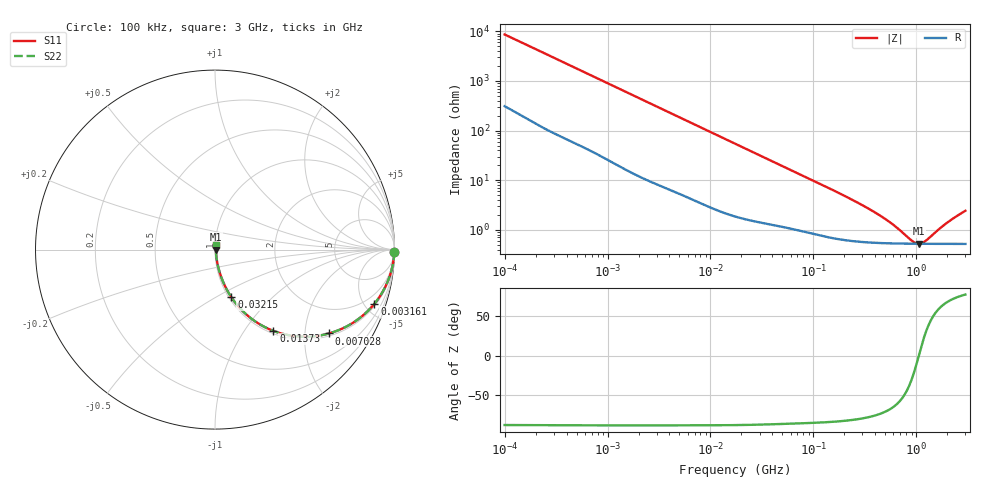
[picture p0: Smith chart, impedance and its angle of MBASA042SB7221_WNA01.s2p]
! MBASA042SB7221_WNA01  S-PARAMETER MODEL  ( Standard Model )
! Model Generated by TAIYO YUDEN Corporation (https://www.yuden.co.jp/en/)
! Version 1.0
! TAIYO YUDEN Control No. 250312
! Copyright(c) 2025 TAIYO YUDEN CO.,LTD. All Rights Reserved.
! Product Description (link to TY-COMPAS)
! https://ds.yuden.co.jp/TYCOMPAS/or/detail?pn=MBASA042SB7221KWNA01&u=M
! Products Name : Multilayer Ceramic Capacitors
! Characteristics :
!  Capacitance : 220 [pF] , Rated Voltage : 4 [V] , TCC : X7R
!  Case Size : 0.4 x 0.2 / 0.016 x 0.008 [mm/inch] , Thickness : 0.2 / 0.008 [mm/inch]
!  (Conditions: Temperature = 25 [degC] , DC Bias Voltage = 0 [V])
! External Node Assignments :
!  1  o---| |---o  2
! GND o---------o GND
! Frequency Range : 100kHz  -  3GHz  [ 401 STEP ]
# MHZ S RI R 50
! Freq[MHz].  S11 Real  S11 Imag  S21 Real  S21 Imag  S12 Real  S12 Imag  S22 Real  S22 Imag
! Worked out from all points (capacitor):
!   401 points, 100 kHz to 3 GHz, reference 50 ohm
!   read as one part in series: C = 183 pF near 105.3 kHz
!   lowest |Z| = 522 mohm at 1.07 GHz (marker M1)
!   series resonance near 1.058 GHz, so ESL is about 120 pH
!   S11 on the Smith chart (normalised r, x): 100 kHz: open; 3.161 MHz: 1.16, -5.83; 7.028 MHz: 1.08, -2.66; 13.73 MHz: 1.04, -1.37; 32.15 MHz: 1.03, -0.59; 3 GHz: 1.01, +0.05
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0.1  0.9995 -0.0115  0.000546 0.0115  0.000546 0.0115  0.9995 -0.0115
0.562235  0.9942 -0.0622  0.00577 0.0622  0.00577 0.0622  0.9942 -0.0622
1.385689  0.9736 -0.1473  0.0264 0.1473  0.0264 0.1473  0.9736 -0.1473
2.203618  0.9402 -0.2243  0.0598 0.2243  0.0598 0.2243  0.9402 -0.2243
3.161081  0.8885 -0.3016  0.1115 0.3016  0.1115 0.3016  0.8885 -0.3016
4.652942  0.7926 -0.3916  0.2074 0.3916  0.2074 0.3916  0.7926 -0.3916
7.027689  0.6352 -0.467  0.3648 0.467  0.3648 0.467  0.6352 -0.467
9.824692  0.4785 -0.4849  0.5215 0.4849  0.5215 0.4849  0.4785 -0.4849
13.7349  0.3258 -0.4532  0.6742 0.4532  0.6742 0.4532  0.3258 -0.4532
17.7727  0.2287 -0.4032  0.7713 0.4032  0.7713 0.4032  0.2287 -0.4032
23.59795  0.1489 -0.337  0.8511 0.337  0.8511 0.337  0.1489 -0.337
32.15051  0.0912 -0.2658  0.9088 0.2658  0.9088 0.2658  0.0912 -0.2658
55.23785  0.0394 -0.1658  0.9606 0.1658  0.9606 0.1658  0.0394 -0.1658
97.38194  0.0179 -0.0975  0.9821 0.0975  0.9821 0.0975  0.0179 -0.0975
287.4592  0.00669 -0.0319  0.9933 0.0319  0.9933 0.0319  0.00669 -0.0319
547.5153  0.00547 -0.0133  0.9945 0.0133  0.9945 0.0133  0.00547 -0.0133
916.7529  0.00521 -0.0027  0.9948 0.0027  0.9948 0.0027  0.00521 -0.0027
990.4458  0.0052 -0.00123  0.9948 0.00123  0.9948 0.00123  0.0052 -0.00123
1070.062  0.00519 0.000221  0.9948 -0.000221  0.9948 -0.000221  0.00519 0.000221
1217.231  0.00519 0.00265  0.9948 -0.00265  0.9948 -0.00265  0.00519 0.00265
1986.261  0.00532 0.0127  0.9947 -0.0127  0.9947 -0.0127  0.00532 0.0127
3000  0.0057 0.0233  0.9943 -0.0233  0.9943 -0.0233  0.0057 0.0233
